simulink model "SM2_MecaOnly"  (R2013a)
settings: Solver=ode23tb  StartTime=0  StopTime=0.1  FixedStep=1e-4  MaxStep=0.5e-3  RelTol=1e-3  AbsTol=1e-4
PreLoadFcn:
  | warning('off','sm:sli:setup:compile:LocalSolverNotSupported')
InitFcn:
  | if(~Model.ModelUpdate)
  |  [~]=SM2_MecaOnly_ConstrFnc(0,Model);
  |  SimParam.IC = SM2_InitCondConstrFnc(RawParam,IC);
  |  Model.ModelUpdate=1;
  | end
model workspace (MAT data in the model file):
  handle : class17 (value not decoded)
  handle : class17 (value not decoded)
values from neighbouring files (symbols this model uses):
  RawParam = RobotParamGather(ParamLib)    [DeltaModelMain_v2.m]    (also in main_TimeSimulation.m; MGI.m = y)
libraries: SM2_BallJointPartsLib x6, SM2_ForeArmPartsLib x6, SM2_ArmPartsLib x3, SM2_MotorPartsLib x3, SM2_FramePartsLib x1, SM2_ToolPartsLib x1

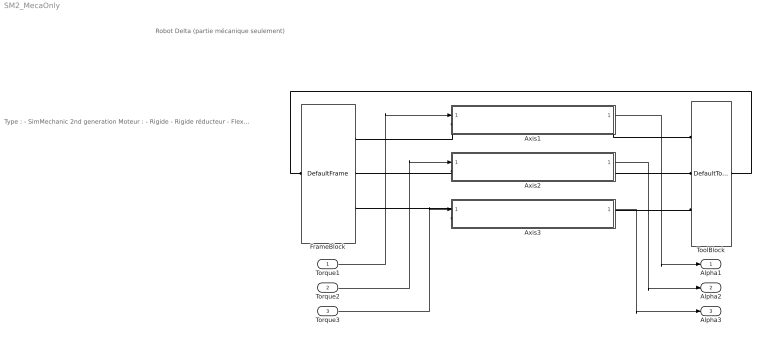
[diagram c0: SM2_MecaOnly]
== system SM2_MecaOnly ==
  note: Robot Delta (partie mécanique seulement)
  note: Type : - SimMechanic 2nd generation Moteur : - Rigide - Rigide réducteur - Flexible 1ddl Bras : - Rigide - Flexible 3ddl (2,3,4 seg.) Rotules - Lineaire (rotule/cardan) AvantBras : - Rigide - Flexible 2ddl (2,3,4,5,6,7 seg.)
  Torque1 : Inport
  Torque2 : Inport  Port=2
  Torque3 : Inport  Port=3
  Axis1 : Subsystem
  Axis2 : Subsystem
  Axis3 : Subsystem
  FrameBlock : SM2_FramePartsLib/DefaultFrame
  ToolBlock : SM2_ToolPartsLib/DefaultTool
  Alpha1 : Outport
  Alpha2 : Outport  Port=2
  Alpha3 : Outport  Port=3
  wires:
  Torque2/1 -> Axis2/1(Torque)
  Torque3/1 -> Axis3/1(Torque)
  Axis1/1(Alpha) -> Alpha1/1
  Axis2/1(Alpha) -> Alpha2/1
  Axis3/1(Alpha) -> Alpha3/1
  Torque1/1 -> Axis1/1(Torque)
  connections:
  Axis1/LConn1 -- FrameBlock/RConn1
  Axis2/LConn1 -- FrameBlock/RConn2
  Axis3/LConn1 -- FrameBlock/RConn3
  Axis3/RConn1 -- ToolBlock/RConn3
  Axis2/RConn1 -- ToolBlock/RConn2
  Axis1/RConn1 -- ToolBlock/RConn1
  FrameBlock/LConn1 -- ToolBlock/LConn1

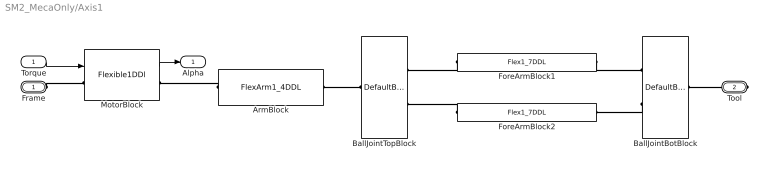
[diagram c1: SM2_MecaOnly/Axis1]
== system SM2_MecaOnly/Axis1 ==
  Torque : Inport
  ArmBlock : SM2_ArmPartsLib/FlexArm1_4DDL  VariantControl=armVarFlex1_4ddl
  BallJointBotBlock : SM2_BallJointPartsLib/DefaultBallJointBotPair
  BallJointTopBlock : SM2_BallJointPartsLib/DefaultBallJointTopPair
  ForeArmBlock1 : SM2_ForeArmPartsLib/Flex1_7DDL  VariantControl=foreArmVarFlex1_7ddl
  ForeArmBlock2 : SM2_ForeArmPartsLib/Flex1_7DDL  VariantControl=foreArmVarFlex1_7ddl
  MotorBlock : SM2_MotorPartsLib/Flexible1DDl  VariantControl=motorVarFlex1
  Frame : PMIOPort  Port=1  Side=Left
  Tool : PMIOPort  Port=2  Side=Right
  Alpha : Outport
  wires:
  Torque/1 -> MotorBlock/1
  MotorBlock/1 -> Alpha/1
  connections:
  ArmBlock/LConn1 -- MotorBlock/RConn1
  Frame/RConn1 -- MotorBlock/LConn1
  BallJointTopBlock/RConn1 -- ArmBlock/RConn1
  Tool/RConn1 -- BallJointBotBlock/RConn1
  ForeArmBlock2/LConn1 -- BallJointTopBlock/LConn2
  ForeArmBlock1/LConn1 -- BallJointTopBlock/LConn1
  ForeArmBlock1/RConn1 -- BallJointBotBlock/LConn1
  BallJointBotBlock/LConn2 -- ForeArmBlock2/RConn1

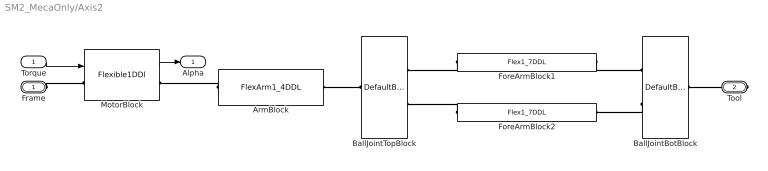
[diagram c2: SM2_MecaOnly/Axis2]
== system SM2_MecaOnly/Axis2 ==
  Torque : Inport
  ArmBlock : SM2_ArmPartsLib/FlexArm1_4DDL  VariantControl=armVarFlex1_4ddl
  BallJointBotBlock : SM2_BallJointPartsLib/DefaultBallJointBotPair
  BallJointTopBlock : SM2_BallJointPartsLib/DefaultBallJointTopPair
  ForeArmBlock1 : SM2_ForeArmPartsLib/Flex1_7DDL  VariantControl=foreArmVarFlex1_7ddl
  ForeArmBlock2 : SM2_ForeArmPartsLib/Flex1_7DDL  VariantControl=foreArmVarFlex1_7ddl
  MotorBlock : SM2_MotorPartsLib/Flexible1DDl  VariantControl=motorVarFlex1
  Frame : PMIOPort  Port=1  Side=Left
  Tool : PMIOPort  Port=2  Side=Right
  Alpha : Outport
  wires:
  Torque/1 -> MotorBlock/1
  MotorBlock/1 -> Alpha/1
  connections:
  ArmBlock/LConn1 -- MotorBlock/RConn1
  Frame/RConn1 -- MotorBlock/LConn1
  BallJointTopBlock/RConn1 -- ArmBlock/RConn1
  Tool/RConn1 -- BallJointBotBlock/RConn1
  ForeArmBlock2/LConn1 -- BallJointTopBlock/LConn2
  ForeArmBlock1/LConn1 -- BallJointTopBlock/LConn1
  ForeArmBlock1/RConn1 -- BallJointBotBlock/LConn1
  BallJointBotBlock/LConn2 -- ForeArmBlock2/RConn1

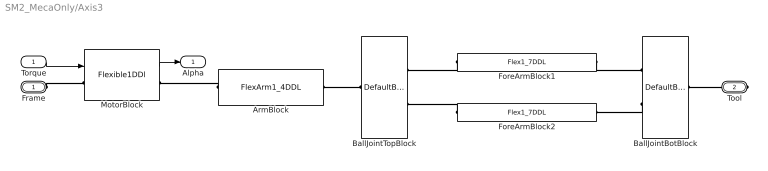
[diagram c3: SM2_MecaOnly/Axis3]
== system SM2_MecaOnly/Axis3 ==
  Torque : Inport
  ArmBlock : SM2_ArmPartsLib/FlexArm1_4DDL  VariantControl=armVarFlex1_4ddl
  BallJointBotBlock : SM2_BallJointPartsLib/DefaultBallJointBotPair
  BallJointTopBlock : SM2_BallJointPartsLib/DefaultBallJointTopPair
  ForeArmBlock1 : SM2_ForeArmPartsLib/Flex1_7DDL  VariantControl=foreArmVarFlex1_7ddl
  ForeArmBlock2 : SM2_ForeArmPartsLib/Flex1_7DDL  VariantControl=foreArmVarFlex1_7ddl
  MotorBlock : SM2_MotorPartsLib/Flexible1DDl  VariantControl=motorVarFlex1
  Frame : PMIOPort  Port=1  Side=Left
  Tool : PMIOPort  Port=2  Side=Right
  Alpha : Outport
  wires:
  Torque/1 -> MotorBlock/1
  MotorBlock/1 -> Alpha/1
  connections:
  ArmBlock/LConn1 -- MotorBlock/RConn1
  Frame/RConn1 -- MotorBlock/LConn1
  BallJointTopBlock/RConn1 -- ArmBlock/RConn1
  Tool/RConn1 -- BallJointBotBlock/RConn1
  ForeArmBlock2/LConn1 -- BallJointTopBlock/LConn2
  ForeArmBlock1/LConn1 -- BallJointTopBlock/LConn1
  ForeArmBlock1/RConn1 -- BallJointBotBlock/LConn1
  BallJointBotBlock/LConn2 -- ForeArmBlock2/RConn1
